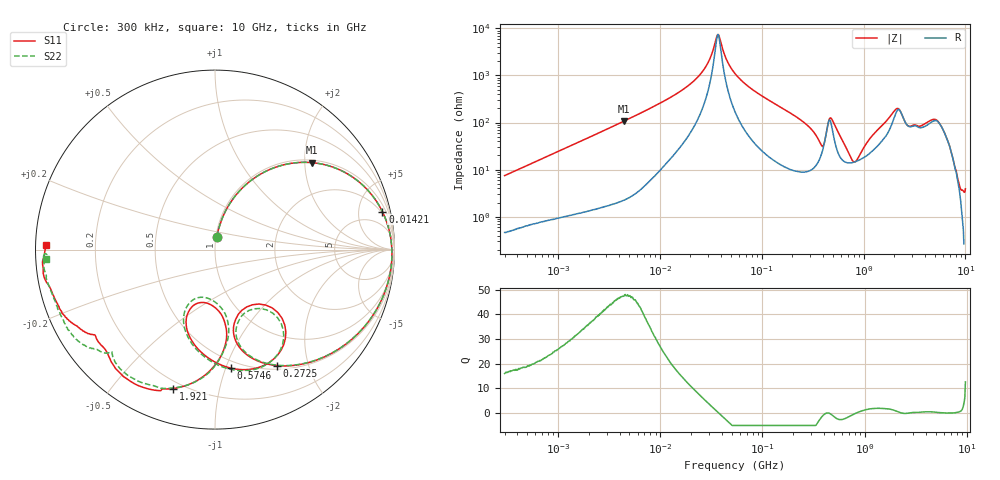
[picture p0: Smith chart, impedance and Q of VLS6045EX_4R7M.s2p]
! S-Parameter Data Generated by TDK Corporation
! Copyright(C) 2019 TDK Corporation.
! All Rights Reserved.
! TDK P/N: VLS6045EX-4R7M (Inductor)
! Property: L=4.7uH at 100kHz
! Size(LxWxT): 6x6x4.5mm
! Model Type: s2p (Touchstone File Format Version 1.0)
! Frequency: DC=Yes Start=0.3MHz Stop=10000MHz 802points Log-sweep
! Model Generated on May 10, 2019
! Port Assignments:
!  1 ---@@@--- 2
! Applicable Conditions:
!  Temperature = 25 degC
!  DC Bias Current = 0 A
!  Small Signal Operation
! Terms and conditions regarding TDK Simulation Models
! (1)This simulation model is being provided solely for informational purposes. Please refer to the specifications of the products in terms of detailed characteristics of such products.
! (2)In no event shall TDK Corporation of any of its subsidiaries be liable for any loss or damage arising, directly or indirectly,
!  From any information contained in this simulation model, including, but not limited to loss or damages arising from any inaccuracies, omissions or errors in connection with such information.
! (3)Any and all copyrights on this simulation model are owned by TDK Corporation.
!  Duplication or redistribution of this simulation model without prior written permission from TDK Corporation is prohibited.
! (4)This simulation model is subject to any modification or change without any prior notice.
! (5)Neither TDK Corporation nor any of its subsidiaries shall make any warranty, express or implied,
!  Including but not limited to the correctness, implied warranties of merchantability and fitness for a particular purpose with respect to this simulation models.
! (6)The use of this simulation model shall be deemed to have consented to the terms and conditions hereof.
# Hz S MA R 50
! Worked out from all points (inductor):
!   801 points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, 300 kHz to 10 GHz, reference 50 ohm
!   read as one part in series: L = 3.93 uH near 318.3 kHz
!   highest Q = 47.5 at 4.487 MHz (marker M1), where L = 3.83 uH
!   self-resonance near 37.3 MHz
!   S11 on the Smith chart (normalised r, x): 300 kHz: 1.01, +0.15; 14.21 MHz: 1.73, +8.57; 272.5 MHz: 0.55, -1.52; 574.6 MHz: 0.44, -1.04; 1.921 GHz: 0.16, -0.73; 10 GHz: 0.03, +0.01
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300000  0.07282 82.2  0.9926 -4.3  0.9929 -4.3  0.07271 81.9
1713600  0.375 66.1  0.9158 -22.2  0.9161 -22.2  0.3749 66.1
4487199  0.7253 41.9  0.6734 -46.9  0.6735 -46.9  0.7253 41.9
9671944  0.9149 21.0  0.3722 -67.0  0.3721 -67.0  0.9149 21.0
1.421446e7  0.9562 12.8  0.2431 -73.9  0.2431 -73.9  0.9563 12.8
2.630692e7  0.9833 2.3  0.0808 -78.1  0.08082 -78.1  0.9833 2.3
3.729897e7  0.9866 -3.2  0.01328 -3.9  0.01329 -3.9  0.9866 -3.2
5.477226e7  0.9822 -9.8  0.08894 71.4  0.08896 71.4  0.9824 -9.7
1.30774e8  0.9211 -31.1  0.338 55.6  0.338 55.6  0.9215 -30.9
2.725454e8  0.7315 -62.0  0.6246 23.6  0.6246 23.6  0.7325 -61.6
3.126428e8  0.658 -69.6  0.6821 14.4  0.6821 14.4  0.6601 -69.0
4.269249e8  0.3895 -51.1  0.6162 -25.0  0.6162 -25.0  0.4144 -52.3
4.74732e8  0.6542 -54.2  0.4027 -12.1  0.4027 -12.1  0.6647 -56.6
5.745924e8  0.6658 -82.5  0.6055 -5.8  0.6054 -5.8  0.6642 -84.4
8.070667e8  0.4986 -107.0  0.7279 -34.5  0.7279 -34.5  0.4847 -109.8
1.149233e9  0.3022 -103.0  0.6846 -73.4  0.6849 -73.4  0.2732 -99.4
1.767019e9  0.7367 -97.8  0.289 -136.8  0.2899 -136.8  0.7336 -97.3
1.920785e9  0.8085 -106.8  0.1945 -141.5  0.1954 -141.5  0.8075 -107.2
2.23379e9  0.8717 -121.0  0.1072 -117.4  0.1079 -117.8  0.8529 -124.2
3.640519e9  0.8247 -144.9  0.113 -137.6  0.1122 -137.7  0.8673 -140.4
5.364878e9  0.9188 -156.8  0.04071 -145.6  0.0404 -145.3  0.9334 -154.2
1e10  0.9405 178.3  0.03588 -141.5  0.03628 -141.2  0.9411 -176.7
